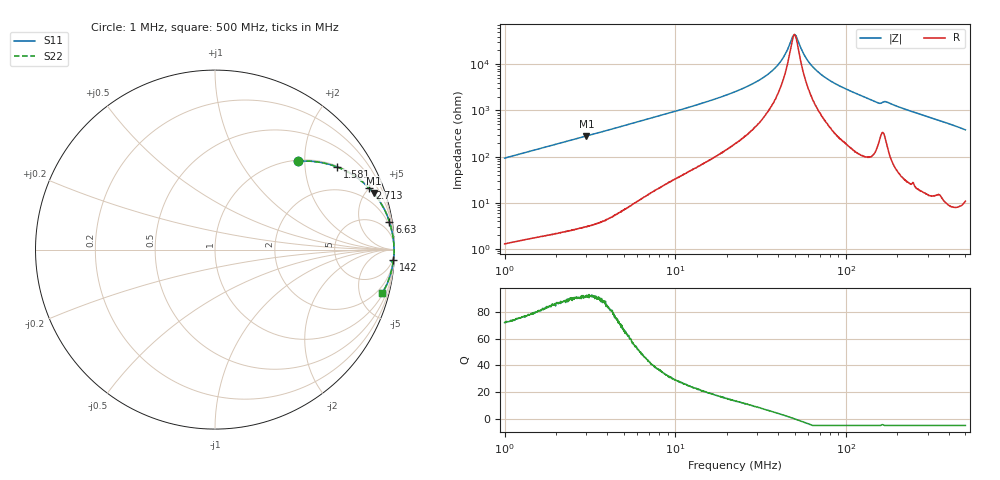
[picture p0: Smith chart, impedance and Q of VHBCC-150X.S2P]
!s-Parameter Generated by FASTRON Sdn. Bhd.
!FASTRON P/N : VHBCC-150X
!Keysight Technologies,E4991B,MY54100416,A.01.15
!Date: Mon Mar 16 11:54:46 2026
!Version  : Rev00 Mon Mar 16 11:54:46 2026
!Data & Calibration Information:
!PortZ  Port1:50+j0  Port2:50+j0
!When reading, reference impedance value at option line is always used.
!Remarks : This data is being provided solely for informational purposes.
!Freq	S11	S21	S12	S22
# Hz S dB R 50
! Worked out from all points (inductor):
!   1601 points, 1 MHz to 500 MHz, reference 50 ohm
!   read as one part in series: L = 14.7 uH near 1.032 MHz
!   highest Q = 92.4 at 3.013 MHz (marker M1), where L = 14.7 uH
!   self-resonance near 49.77 MHz
!   S11 on the Smith chart (normalised r, x): 1 MHz: 1.03, +1.86; 1.581 MHz: 1.04, +2.93; 2.713 MHz: 1.06, +5.02; 6.63 MHz: 1, +12; 142 MHz: 3, -33; 500 MHz: 1.22, -7.61
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1000000  -3.41 46.7  -2.76 -42.5  -2.76 -42.5  -3.41 46.7
1581427  -1.71 34.1  -5.02 -55.2  -5.02 -55.2  -1.71 34.1
2713451  -0.67 21.6  -8.67 -67.7  -8.67 -67.7  -0.67 21.6
2820919  -0.63 20.9  -8.96 -68.5  -8.96 -68.5  -0.63 20.9
3013472  -0.55 19.7  -9.47 -69.7  -9.47 -69.7  -0.55 19.7
6629778  -0.14 9.1  -16.06 -79.7  -16.06 -79.7  -0.14 9.1
7957584  -0.11 7.5  -17.67 -81.0  -17.67 -81.0  -0.11 7.5
2.236068e7  -0.03 2.2  -28.15 -83.5  -28.15 -83.5  -0.03 2.2
3.050939e7  -0.03 1.3  -32.88 -82.0  -32.88 -82.0  -0.03 1.3
3.762909e7  -0.02 0.7  -37.80 -78.2  -37.80 -78.2  -0.02 0.7
4.2775e7  -0.02 0.4  -42.84 -70.2  -42.84 -70.2  -0.02 0.4
4.843613e7  -0.02 0.1  -51.62 -29.1  -51.62 -29.1  -0.02 0.1
4.977112e7  -0.02 0.0  -52.96 -1.8  -52.96 -1.8  -0.02 0.0
5.134194e7  -0.02 -0.1  -51.73 29.8  -51.73 29.8  -0.02 -0.1
5.746337e7  -0.02 -0.4  -43.52 70.2  -43.52 70.2  -0.02 -0.4
6.307767e7  -0.02 -0.6  -39.35 77.7  -39.35 77.7  -0.02 -0.6
7.11489e7  -0.02 -0.9  -35.72 81.3  -35.72 81.3  -0.02 -0.9
8.310792e7  -0.02 -1.4  -32.38 83.6  -32.38 83.6  -0.02 -1.4
1.420459e8  -0.05 -3.4  -24.49 83.1  -24.49 83.1  -0.05 -3.4
1.553196e8  -0.10 -3.9  -23.27 78.2  -23.27 78.2  -0.10 -3.9
1.77937e8  -0.07 -3.9  -23.38 81.4  -23.38 81.4  -0.07 -3.9
5e8  -0.35 -14.6  -11.96 73.8  -11.96 73.8  -0.35 -14.6
